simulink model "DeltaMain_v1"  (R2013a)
settings: Solver=ode23  StartTime=0  StopTime=0.4  FixedStep=1e-4  MaxStep=1e-3  RelTol=1e-3  AbsTol=1e-4
PreLoadFcn:
  | warning('off','sm:sli:setup:compile:LocalSolverNotSupported')
model workspace (MAT data in the model file):
  handle : class17 (value not decoded)
  handle : class17 (value not decoded)
undefined symbols (not defined in the file or in its folder): SimParam

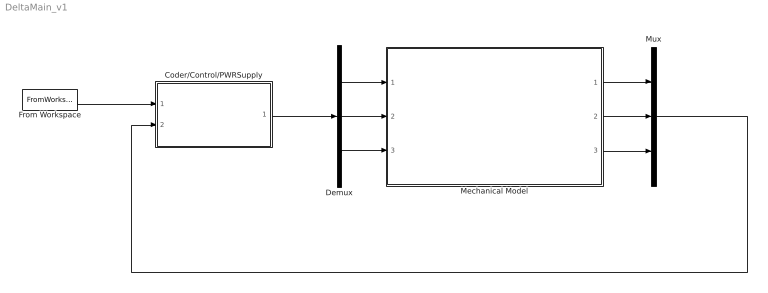
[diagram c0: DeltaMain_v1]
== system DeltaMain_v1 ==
  Coder/Control/PWRSupply : Subsystem
  Demux : Demux  Outputs=3
  From Workspace : FromWorkspace  VariableName=simin  SampleTime=SimParam.Control.Te  OutputAfterFinalValue=Holding final value
  Mechanical Model : ModelReference  ModelNameDialog=MecaOnly_sm1.slx  SimulationMode=Normal  ModelReferenceVersion=1.395  CopyOfModelName=MecaOnly_sm1.slx  DefaultDataLogging=on
  Mux : Mux  Inputs=3
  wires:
  Coder/Control/PWRSupply/1(Torque) -> Demux/1
  Mux/1 -> Coder/Control/PWRSupply/2(Alpha)
  Demux/3 -> Mechanical Model/3
  Demux/2 -> Mechanical Model/2
  Demux/1 -> Mechanical Model/1
  Mechanical Model/3 -> Mux/3
  Mechanical Model/2 -> Mux/2
  Mechanical Model/1 -> Mux/1
  From Workspace/1 -> Coder/Control/PWRSupply/1(Alpha_c)

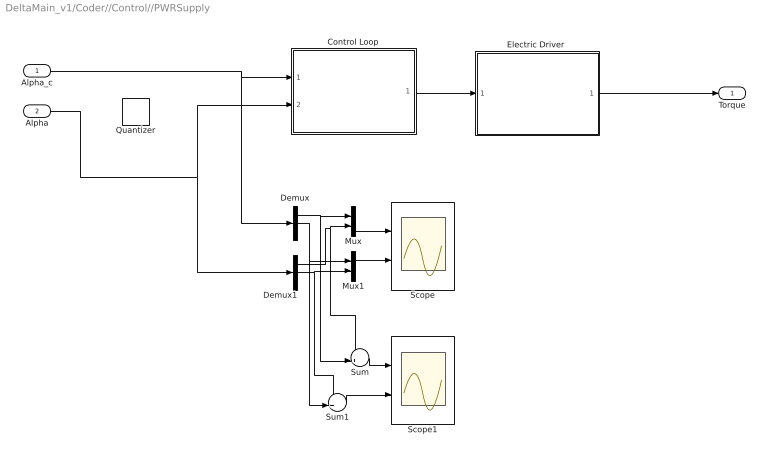
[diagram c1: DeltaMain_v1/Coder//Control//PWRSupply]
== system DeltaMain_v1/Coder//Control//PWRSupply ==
  Alpha_c : Inport
  Alpha : Inport  Port=2
  Control Loop : Subsystem  Variant=on
  Demux : Demux  Outputs=3
  Demux1 : Demux  Outputs=3
  "Electric Driver " : Subsystem  Variant=on
  Mux : Mux  Inputs=2
  Mux1 : Mux  Inputs=2
  Quantizer : Quantizer  Commented=on  QuantizationInterval=7e-5
  Scope : Scope  NumInputPorts=2
  Scope1 : Scope  NumInputPorts=2
  Sum : Sum  Inputs=-+|
  Sum1 : Sum  Inputs=-+|
  Torque : Outport
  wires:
  Control Loop/1(U) -> "Electric Driver "/1(U)
  Alpha_c/1 -> Demux/1, Control Loop/1(Alpha_c)
  Demux/1 -> Sum/2, Mux/1
  Demux1/2 -> Sum1/1, Mux1/2
  Demux/2 -> Sum1/2, Mux1/1
  Mux/1 -> Scope/1
  Mux1/1 -> Scope/2
  "Electric Driver "/1(Torque) -> Torque/1
  Sum/1 -> Scope1/1
  Sum1/1 -> Scope1/2
  Demux1/1 -> Sum/1, Mux/2
  Alpha/1 -> Demux1/1, Control Loop/2(Alpha)

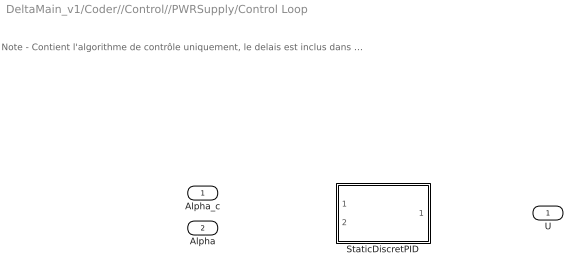
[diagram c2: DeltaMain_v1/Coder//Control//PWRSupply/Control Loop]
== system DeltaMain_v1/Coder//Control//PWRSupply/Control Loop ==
  note: Note - Contient l'algorithme de contrôle uniquement, le delais est inclus dans le bloque 'Electric Drive'
  Alpha_c : Inport
  Alpha : Inport  Port=2
  StaticDiscretPID : Subsystem  VariantControl=controlVarDefault
  U : Outport

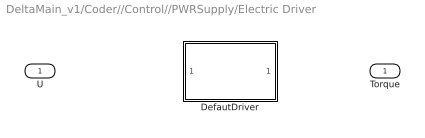
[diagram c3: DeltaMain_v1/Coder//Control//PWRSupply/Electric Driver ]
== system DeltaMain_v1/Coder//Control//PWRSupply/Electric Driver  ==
  U : Inport
  DefautDriver : Subsystem  VariantControl=driverVarDefault
  Torque : Outport

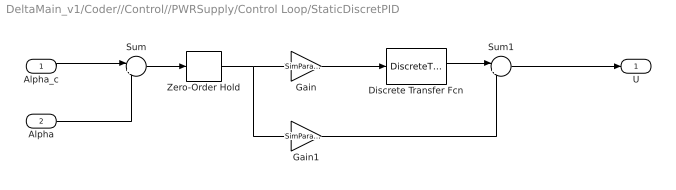
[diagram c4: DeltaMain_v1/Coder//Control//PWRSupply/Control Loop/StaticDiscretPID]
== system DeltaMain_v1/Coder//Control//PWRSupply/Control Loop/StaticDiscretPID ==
  Alpha_c : Inport
  Alpha : Inport  Port=2
  Discrete Transfer Fcn : DiscreteTransferFcn  Numerator=[1 0 -1]  Denominator=[2 0 0]
  Gain : Gain  Gain=SimParam.Control.Kd/SimParam.Control.Te
  Gain1 : Gain  Gain=SimParam.Control.Kp
  Sum : Sum  Inputs=|+-
  Sum1 : Sum  Inputs=|++
  Zero-Order Hold : ZeroOrderHold  SampleTime=SimParam.Control.Te
  U : Outport
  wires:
  Alpha/1 -> Sum/2
  Alpha_c/1 -> Sum/1
  Sum/1 -> Zero-Order Hold/1
  Gain/1 -> Discrete Transfer Fcn/1
  Zero-Order Hold/1 -> Gain/1, Gain1/1
  Gain1/1 -> Sum1/2
  Discrete Transfer Fcn/1 -> Sum1/1
  Sum1/1 -> U/1

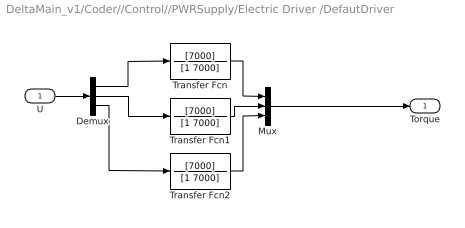
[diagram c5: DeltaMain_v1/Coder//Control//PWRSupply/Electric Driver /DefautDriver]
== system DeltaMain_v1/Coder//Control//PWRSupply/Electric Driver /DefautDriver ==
  U : Inport
  Demux : Demux  Outputs=3
  Mux : Mux  Inputs=3
  Transfer Fcn : TransferFcn  Numerator=[7000]  Denominator=[1 7000]
  Transfer Fcn1 : TransferFcn  Numerator=[7000]  Denominator=[1 7000]
  Transfer Fcn2 : TransferFcn  Numerator=[7000]  Denominator=[1 7000]
  Torque : Outport
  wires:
  U/1 -> Demux/1
  Demux/1 -> Transfer Fcn/1
  Demux/2 -> Transfer Fcn1/1
  Demux/3 -> Transfer Fcn2/1
  Mux/1 -> Torque/1
  Transfer Fcn2/1 -> Mux/3
  Transfer Fcn1/1 -> Mux/2
  Transfer Fcn/1 -> Mux/1
